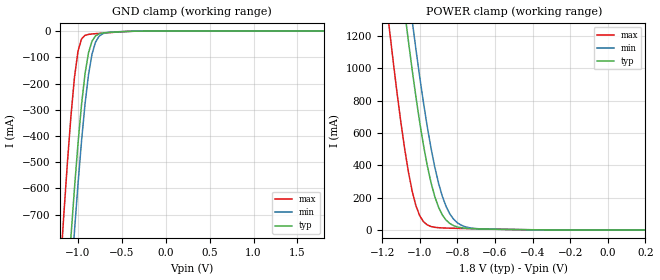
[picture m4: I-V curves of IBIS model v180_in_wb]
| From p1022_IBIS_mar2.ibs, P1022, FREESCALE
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|   Model v180_in_wb
[Model]   v180_in_wb
Model_type   Input
Polarity   Non-Inverting
Enable   Active-High
Vinl = 0.63V
Vinh = 1.17V
C_comp   3.0088pF   2.9071pF   3.0187pF
[Temperature Range]   85.0000   0.1250k   -40.0000
[Voltage Range]   1.8000V   1.6200V   1.9800V
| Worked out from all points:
|   GND clamp passes 1 mA (typ) near -0.40 V on its own axis
|   POWER clamp passes 1 mA (typ) near -0.37 V on its own axis
[GND_clamp]
|Voltage   I(typ)   I(min)   I(max)
-1.8V     -4.804A    -4.965A    -4.352A
-1.2V     -1.391A    -1.566A    -898mA
-1.16V    -1.182A    -1.356A    -692.5mA
-1.08V    -783mA     -952.3mA   -322.2mA
-1.04V    -598.3mA   -762.1mA   -175.8mA
-1V       -428.7mA   -583.2mA   -76.41mA
-920mV    -162.7mA   -278.3mA   -16.12mA
-880mV    -82.2mA    -165.4mA   -12.47mA
-840mV    -37.92mA   -87mA      -10.97mA
-800mV    -18.2mA    -41.64mA   -9.843mA
-720mV    -7.422mA   -10.26mA   -7.766mA
1.8V      9.036uA    41.65uA    11.05uA
[POWER_clamp]
|Voltage   I(typ)   I(min)   I(max)
-1.8V     9.621A     9.869A     8.815A
-1.16V    2.159A     2.491A     1.232A
-1.08V    1.354A     1.674A     501.9mA
-1.06V    1.168A     1.482A     358.5mA
-1.04V    989.9mA    1.296A     239.6mA
-1V       666mA      947mA      88.04mA
-960mV    399.2mA    640.1mA    31.27mA
-920mV    207mA      389.6mA    16.4mA
-880mV    93.61mA    209mA      12.71mA
-840mV    40.16mA    99.64mA    11.19mA
-780mV    13.9mA     30.06mA    9.524mA
200mV     0A         0A         0A
